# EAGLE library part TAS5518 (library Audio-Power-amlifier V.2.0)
The TAS5518 is an eight channel digital pulse width a modulator (PWM) that provides superior dynamic range performance and a high level of system integration. The typical dynamic range in a well-designed system is 110 dB and the power supply volume control (PSVC) feature provides up to 24 dB of additional dynamic range at normal listening levels. The TAS5518 is designed to interface seamlessly with most audio digital signal processors. This device automatically adjusts control configurations in response to clock and data rate changes and idle conditions. This enables the TAS5518 to provide an easy to use control interface with relaxed timing requirements. The TAS5518 can drive eight channels of H-bridge power stages. Texas Instruments H-bridge devices TAS5111, TAS5112, and TAS5182 + FETs are designed to work seamlessly with the TAS5518. The TAS5518 supports both single-ended or bridge-tied load configurations. It also provides a high-performance differential output to drive an external differential input analog headphone amplifier (such as the TPA112). The TAS5518 uses an AD modulation operating at a 384-kHz switching rate for 48-, 96-, and 192-kHz data. The 8x over sampling, combined with a 5th-order noise shaper, provides a broad flat noise floor and excellent dynamic range from 20 Hz to 20 kHz. The TAS5518 is a clock slave-only device. It receives MCLK, SCLK, and LRCLK from other system components. It accepts master clock rates of 128, 192, 256, 384, 512, and 768 Fs and a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
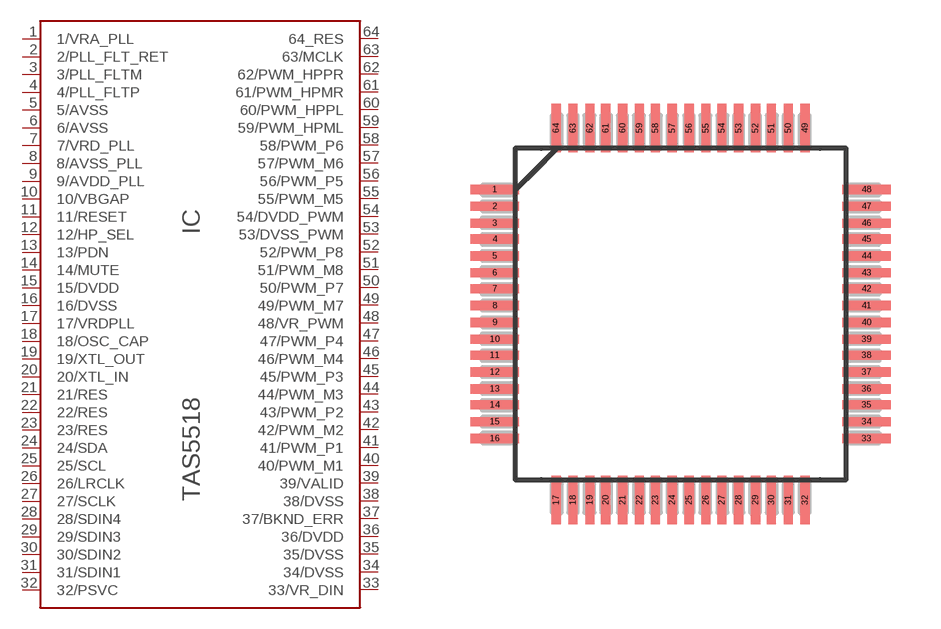
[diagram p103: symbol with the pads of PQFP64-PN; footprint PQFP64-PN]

Designator prefix IC

## TAS5518  [PQFP64-PN]
1  1/VRA_PLL  out
2  2/PLL_FLT_RET
3  3/PLL_FLTM  in
4  4/PLL_FLTP  in
5  5/AVSS  pwr
6  6/AVSS  pwr
7  7/VRD_PLL  out
8  8/AVSS_PLL  pwr
9  9/AVDD_PLL  pwr
10  10/VBGAP  out
11  11/RESET  in
12  12/HP_SEL
13  13/PDN
14  14/MUTE  out
15  15/DVDD  pwr
16  16/DVSS  pwr
17  17/VRDPLL  out
18  18/OSC_CAP  in
19  19/XTL_OUT  out
20  20/XTL_IN  in
21  21/RES  pwr
22  22/RES  pwr
23  23/RES  pwr
24  24/SDA
25  25/SCL
26  26/LRCLK
27  27/SCLK  in
28  28/SDIN4  in
29  29/SDIN3  in
30  30/SDIN2  in
31  31/SDIN1  in
32  32/PSVC  out
33  33/VR_DIN  out
34  34/DVSS  pwr
35  35/DVSS  pwr
36  36/DVDD  pwr
37  37/BKND_ERR
38  38/DVSS  pwr
39  39/VALID  out
40  40/PWM_M1  out
41  41/PWM_P1  out
42  42/PWM_M2  out
43  43/PWM_P2  out
44  44/PWM_M3  out
45  45/PWM_P3  out
46  46/PWM_M4  out
47  47/PWM_P4  out
48  48/VR_PWM  out
49  49/PWM_M7  out
50  50/PWM_P7  out
51  51/PWM_M8  out
52  52/PWM_P8  out
53  53/DVSS_PWM  pwr
54  54/DVDD_PWM  pwr
55  55/PWM_M5  out
56  56/PWM_P5  out
57  57/PWM_M6  out
58  58/PWM_P6  out
59  59/PWM_HPML  out
60  60/PWM_HPPL  out
61  61/PWM_HPMR  out
62  62/PWM_HPPR  out
63  63/MCLK  in
64  64_RES  pwr

## Footprint PQFP64-PN (pad centres in mm)
PAG (S-PQFP-G64)
smd 1.473 x 0.279: 1 -5.613,3.759; 2 -5.613,3.251; 3 -5.613,2.743; 4 -5.613,2.261; 5 -5.613,1.753; 6 -5.613,1.245; 7 -5.613,0.762; 8 -5.613,0.254; 9 -5.613,-0.254; 10 -5.613,-0.762; 11 -5.613,-1.245; 12 -5.613,-1.753; 13 -5.613,-2.261; 14 -5.613,-2.743; 15 -5.613,-3.251; 16 -5.613,-3.759; 33 5.613,-3.759; 34 5.613,-3.251; 35 5.613,-2.743; 36 5.613,-2.261; 37 5.613,-1.753; 38 5.613,-1.245; 39 5.613,-0.762; 40 5.613,-0.254; 41 5.613,0.254; 42 5.613,0.762; 43 5.613,1.245; 44 5.613,1.753; 45 5.613,2.261; 46 5.613,2.743; 47 5.613,3.251; 48 5.613,3.759
smd 0.279 x 1.473: 17 -3.759,-5.613; 18 -3.251,-5.613; 19 -2.743,-5.613; 20 -2.261,-5.613; 21 -1.753,-5.613; 22 -1.245,-5.613; 23 -0.762,-5.613; 24 -0.254,-5.613; 25 0.254,-5.613; 26 0.762,-5.613; 27 1.245,-5.613; 28 1.753,-5.613; 29 2.261,-5.613; 30 2.743,-5.613; 31 3.251,-5.613; 32 3.759,-5.613; 49 3.759,5.613; 50 3.251,5.613; 51 2.743,5.613; 52 2.261,5.613; 53 1.753,5.613; 54 1.245,5.613; 55 0.762,5.613; 56 0.254,5.613; 57 -0.254,5.613; 58 -0.762,5.613; 59 -1.245,5.613; 60 -1.753,5.613; 61 -2.261,5.613; 62 -2.743,5.613; 63 -3.251,5.613; 64 -3.759,5.613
